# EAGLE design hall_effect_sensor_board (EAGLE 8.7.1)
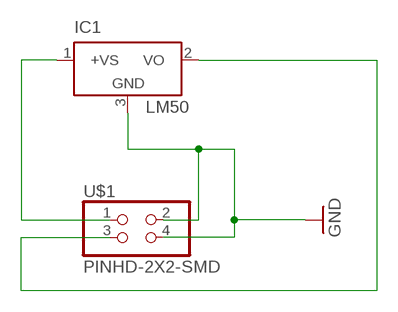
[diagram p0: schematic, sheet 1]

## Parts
IC1  LM50  [SOT23]
U$1  PINHD-2X2-SMD  [2X02SMD]

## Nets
GND: IC1.3(GND) U$1.2 U$1.4
N$1: IC1.1(+VS) U$1.1
N$3: IC1.2(VO) U$1.3

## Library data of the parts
IC1 = linear:LM50: SOT-23 Single-Supply Centigrade Temperature Sensor Vout = (10mV/°C x Temp °C) +5mmmV Source: http://cache.national.com/ds/LM/LM50.pdf
U$1 = fab:PINHD-2X2-SMD

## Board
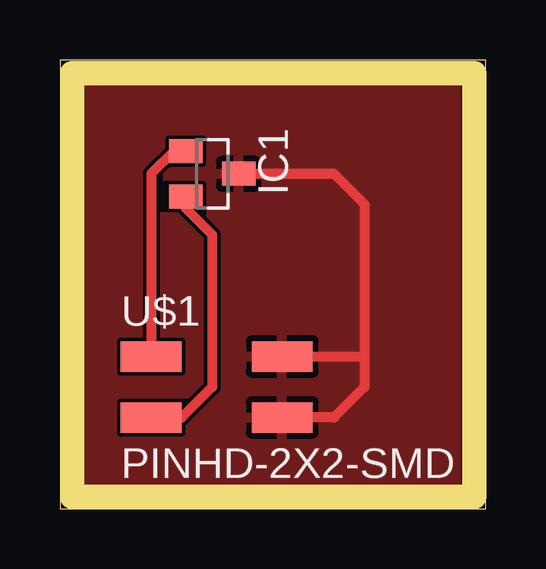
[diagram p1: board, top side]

Size 17.76 x 18.72 mm. Coordinates in mm from the lower left corner, seen from the top.
Outline: 0,0 17.76,0 17.76,18.72 0,18.72 0,0
Copper layers (1*16): Top 0.035mm / dielectric 1.5mm / Bottom 0.035mm
Design rules "default": minimum track width 6mil, minimum drill 0.35mm, track to track 6mil, track to pad 6mil, pad to pad 6mil, via to via 6mil, smd to smd 6mil, copper to edge 40mil, drill to drill 6mil, minimum pad ring 10mil, minimum via ring 8mil, stop-mask expansion 4mil, vias tented up to drill 0mil, thermal gap 10mil
Milling: 4 lines

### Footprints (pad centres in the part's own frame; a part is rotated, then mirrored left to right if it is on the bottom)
SOT23 = smd 1 x 1.4: 1 -0.95,-1.1; 2 0.95,-1.1; 3 0,1.1
2X02SMD = smd 2.54 x 1.27: 1 -2.54,1.27; 2 2.92,1.27; 3 -2.54,-1.27; 4 2.92,-1.27

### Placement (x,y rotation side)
IC1  6.35,13.97 270 top
U$1  6.35,5.08 0 top

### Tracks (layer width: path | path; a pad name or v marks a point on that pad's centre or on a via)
GND
  Top 0.406: IC1.3 11.43,13.97 12.7,12.7 12.7,6.35 | 12.7,6.35 12.7,5.08 11.43,3.81 U$1.4 | U$1.2 12.7,6.35
  pour Top: 0,19.05 17.78,19.05 17.78,0 0,0
N$1
  Top 0.406: IC1.1 4.76,14.92 3.81,13.97 U$1.1
N$3
  Top 0.406: IC1.2 5.25,12.53 6.35,11.43 6.35,5.08 5.08,3.81 U$1.3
